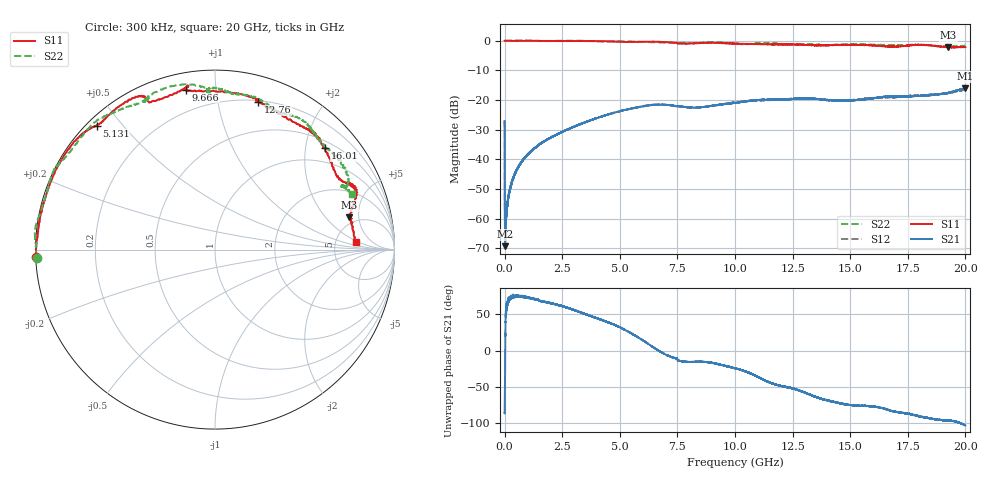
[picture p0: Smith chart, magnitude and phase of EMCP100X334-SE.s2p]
!EMCP100X334
!Johanson Technology Inc.
!www.johansontechnology.com
!Test Board Conditions:
!Substrate Type  RO4350B
!Substrate Thickness  10 mil
!Substrate Dk  3.66
!TL Type: GCPW
!TL Trace Width  20 mil
!TL Gap  10 mil
!PART MODE SINGLE ENDED (AKA BYPASS)
!DUT TOPOLOGY	SERIES-SHUNT
# MHz S  dB  R 50
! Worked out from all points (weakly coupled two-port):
!   20001 points, 300 kHz to 20 GHz, reference 50 ohm
!   highest |S21| = -16.11 dB at 19.98 GHz (marker M1); lowest = -69.3 dB at 24.3 MHz (marker M2)
!   lowest |S11| = -2.3 dB at 19.27 GHz (marker M3), VSWR 7.72, Z = 213 + j189 ohm
!   |S11| at or under -10 dB: nowhere
!   |S22| runs from -2.1 to 0.1 dB; largest |S21 - S12| = 0.0078
!   S11 on the Smith chart (normalised r, x): 300 kHz: 0.00, -0.02; 5.131 GHz: 0.03, +0.43; 9.666 GHz: 0.08, +0.83; 12.76 GHz: 0.21, +1.31; 16.01 GHz: 0.65, +2.41; 20 GHz: 7.89, +1.67
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0.3  -0.03 -177.7  -27.11 -86.1  -27.03 -85.9  -0.04 -177.3
24.3  -0.02 179.8  -69.33 -13.6  -68.10 -10.4  -0.03 179.9
105.298  -0.03 178.8  -57.00 63.0  -56.40 59.5  -0.04 179.3
215.297  -0.04 177.8  -50.76 70.2  -50.95 73.2  -0.03 178.4
369.294  -0.07 176.0  -46.42 73.5  -46.43 73.2  0.02 177.3
907.286  -0.07 170.8  -39.20 73.3  -39.20 73.5  0.07 172.7
1747.274  -0.09 166.7  -33.86 66.9  -33.79 66.9  -0.09 162.6
3334.25  -0.08 148.3  -27.98 52.0  -27.99 52.4  -0.03 151.9
5131.223  -0.40 133.7  -23.53 30.1  -23.57 30.1  -0.22 135.7
6667.2  -0.37 117.5  -21.58 0.2  -21.52 -0.1  -0.57 122.9
8638.17  -0.73 99.9  -22.36 -15.5  -22.37 -16.1  -0.67 113.8
9666.155  -0.86 100.4  -21.29 -21.9  -21.19 -21.0  -0.76 95.3
10000.15  -0.99 98.4  -20.97 -24.3  -20.78 -24.2  -1.00 92.5
11336.13  -1.18 75.3  -19.92 -41.6  -20.04 -41.4  -0.92 90.9
12762.11  -1.35 73.8  -19.56 -54.8  -19.49 -55.0  -1.14 78.8
13334.1  -1.52 66.9  -19.52 -61.9  -19.49 -62.2  -1.26 72.0
16013.06  -1.58 42.6  -19.38 -77.1  -19.29 -78.9  -1.37 50.2
16667.05  -1.99 33.3  -18.81 -81.9  -19.07 -82.0  -1.47 47.0
18125.03  -1.40 22.8  -18.60 -91.2  -18.37 -91.6  -1.47 29.8
19266.01  -2.26 13.5  -17.59 -96.2  -17.71 -97.8  -2.10 26.6
19983  -2.12 3.0  -16.11 -102.7  -16.47 -101.0  -1.66 22.3
20000  -2.12 3.0  -16.16 -103.1  -16.41 -101.1  -1.67 22.2
